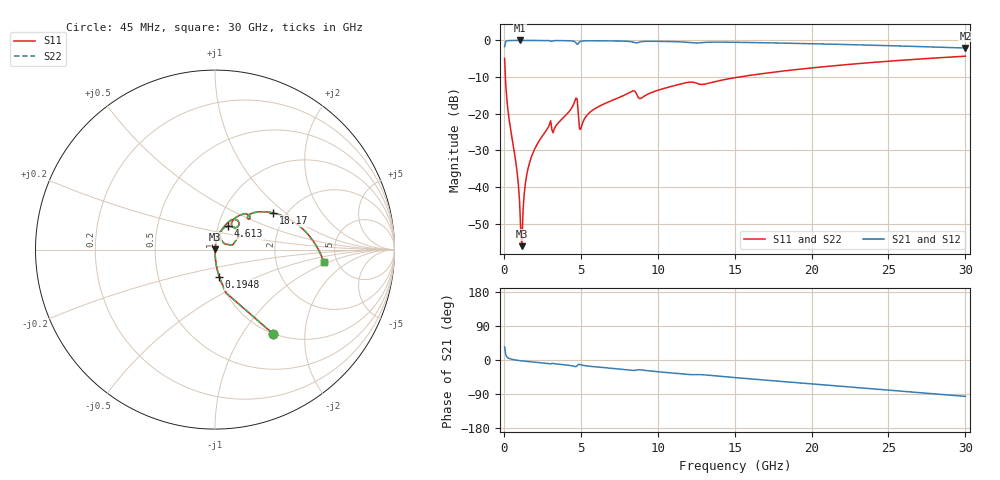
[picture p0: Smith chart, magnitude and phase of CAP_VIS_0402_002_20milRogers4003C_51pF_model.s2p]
! S-parameter model data by Modelithics Inc.  support@modelithics.com  813-866-6335  Tampa FL USA
! S-Parameter data specifications:
! Substrate: 20-mil Rogers 4003C, substrate thickness, H=0.508mm, Dielectric constant, Er=3.75
! PCB Mounting Pad Footprint: Pad width, PadW=0.50mm , Pad length, PadL=0.50mm , Pad gap, PadG (edge-to-edge)=0.40mm , Reference planes=1.4mm apart
! Created Wed Nov 18 12:55:39 2015
# hz S ma R 50
! 2 Port Network Data from SP1.SP block
! freq  magS11  angS11  magS21  angS21  magS12  angS12  magS22  angS22
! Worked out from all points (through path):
!   401 points, 45 MHz to 30 GHz, reference 50 ohm
!   highest |S21| = -0.01 dB at 1.019 GHz (marker M1); lowest = -2.1 dB at 30 GHz (marker M2)
!   group delay of S21, straight-line fit = 9.02 ps
!   lowest |S11| = -56.2 dB at 1.168 GHz (marker M3), VSWR 1.00, Z = 50.1 + j0.122 ohm
!   |S11| at or under -10 dB: 98.02 MHz to 15.28 GHz (15.18 GHz wide, 197 % of centre)
!   |S22| runs from -56.2 to -4.3 dB; largest |S21 - S12| = 0
!   S11 on the Smith chart (normalised r, x): 45 MHz: 1.00, -1.38; 194.8 MHz: 1.00, -0.31; 4.613 GHz: 1.11, +0.30; 18.17 GHz: 1.71, +0.82; 30 GHz: 3.92, -0.85
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4.5e7  0.5678 -55.5  0.823 34.5  0.823 34.5  0.5678 -55.5
1.94775e8  0.1531 -81.4  0.9878 8.4  0.9878 8.4  0.1531 -81.4
3.4455e8  0.08176 -85.6  0.9961 4.0  0.9961 4.0  0.08176 -85.6
7.93875e8  0.02029 -88.2  0.999 -0.3  0.999 -0.3  0.02029 -88.2
1.018538e9  0.006323 -83.8  0.9991 -1.6  0.9991 -1.6  0.006323 -83.8
1.168312e9  0.001551 51.6  0.999 -2.3  0.999 -2.3  0.001551 51.6
1.2432e9  0.004761 76.0  0.999 -2.6  0.999 -2.6  0.004761 76.0
1.54275e9  0.01686 82.5  0.9988 -3.9  0.9988 -3.9  0.01686 82.5
1.992075e9  0.03264 82.2  0.9982 -5.6  0.9982 -5.6  0.03264 82.2
2.890725e9  0.06586 78.1  0.9947 -9.2  0.9947 -9.2  0.06586 78.1
3.265162e9  0.06132 76.3  0.9937 -9.7  0.9937 -9.7  0.06132 76.3
4.613138e9  0.149 61.1  0.9588 -17.1  0.9588 -17.1  0.149 61.1
5.062462e9  0.0687 62.6  0.9809 -13.4  0.9809 -13.4  0.0687 62.6
6.560212e9  0.1374 68.4  0.9872 -20.3  0.9872 -20.3  0.1374 68.4
8.357512e9  0.2036 55.3  0.9534 -27.4  0.9534 -27.4  0.2036 55.3
8.881725e9  0.1612 53.4  0.9571 -25.9  0.9571 -25.9  0.1612 53.4
1.007992e10  0.2109 57.2  0.9714 -31.2  0.9714 -31.2  0.2109 57.2
1.50225e10  0.3098 42.3  0.9437 -46.5  0.9437 -46.5  0.3098 42.3
1.816778e10  0.3822 32.3  0.9188 -57.0  0.9188 -57.0  0.3822 32.3
2.003996e10  0.4219 26.3  0.9015 -63.1  0.9015 -63.1  0.4219 26.3
2.505742e10  0.5213 9.9  0.8479 -79.6  0.8479 -79.6  0.5213 9.9
3e10  0.6095 -6.4  0.7867 -96.0  0.7867 -96.0  0.6095 -6.4
